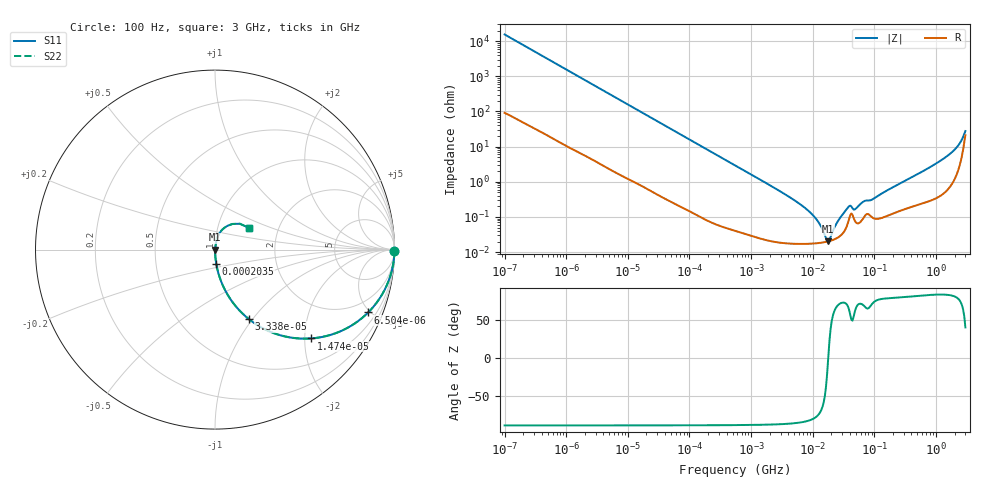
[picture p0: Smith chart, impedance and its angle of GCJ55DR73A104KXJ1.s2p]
!Murata Part Number: GCJ55DR73A104KXJ1
!These Parameters are Measured in Series Mode Connection
!Data Generated on Mar 13, 2026
!  o--ll--o
!Port1  Port2
!  o------o
!Operation Temp=25[degC], DC Bias Voltage=0[V]
!Freq. Start=100[Hz] Stop=3[GHz] 401[Steps]
# Hz S RI R 50
!Freq.(Hz) S11(Real) S11(Imag) S21(Real) S21(Imag) S12(Real) S12(Imag) S22(Real) S22(Imag)
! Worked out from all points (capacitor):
!   401 points, 100 Hz to 3 GHz, reference 50 ohm
!   read as one part in series: C = 103 nF near 109 Hz
!   lowest |Z| = 20.2 mohm at 17.89 MHz (marker M1)
!   series resonance near 17.83 MHz, so ESL is about 780 pH
!   S11 on the Smith chart (normalised r, x): 100 Hz: open; 6.504 kHz: 1.04, -4.86; 14.74 kHz: 1.02, -2.15; 33.38 kHz: 1.01, -0.95; 203.5 kHz: 1.00, -0.16; 3 GHz: 1.42, +0.36
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100  0.9999 -0.00645  7.96e-05 0.00645  7.96e-05 0.00645  0.9999 -0.00645
1788  0.9864 -0.1123  0.0136 0.1123  0.0136 0.1123  0.9864 -0.1123
6504  0.8532 -0.3503  0.1468 0.3503  0.1468 0.3503  0.8532 -0.3503
14736  0.5363 -0.4947  0.4637 0.4947  0.4637 0.4947  0.5363 -0.4947
31977  0.2006 -0.3964  0.7994 0.3964  0.7994 0.3964  0.2006 -0.3964
33383  0.1874 -0.3861  0.8126 0.3861  0.8126 0.3861  0.1874 -0.3861
69391  0.0521 -0.2179  0.9479 0.2179  0.9479 0.2179  0.0521 -0.2179
203529  0.00694 -0.0784  0.9931 0.0784  0.9931 0.0784  0.00694 -0.0784
547723  0.00127 -0.0294  0.9987 0.0294  0.9987 0.0294  0.00127 -0.0294
4323298  0.000187 -0.00355  0.9998 0.00355  0.9998 0.00355  0.000187 -0.00355
9794414  0.000176 -0.00117  0.9998 0.00117  0.9998 0.00117  0.000176 -0.00117
1.268047e7  0.000182 -0.000642  0.9998 0.000642  0.9998 0.000642  0.000182 -0.000642
1.789277e7  0.000202 6.4e-06  0.9998 -6.4e-06  0.9998 -6.4e-06  0.000202 6.4e-06
2.635803e7  0.000269 0.000778  0.9997 -0.000778  0.9997 -0.000778  0.000269 0.000778
3.71925e7  0.000674 0.00172  0.9993 -0.00172  0.9993 -0.00172  0.000674 0.00172
5.026954e7  0.000697 0.00159  0.9993 -0.00159  0.9993 -0.00159  0.000697 0.00159
6.794454e7  0.000996 0.00261  0.999 -0.00261  0.999 -0.00261  0.000996 0.00261
9.183415e7  0.000985 0.00296  0.999 -0.00296  0.999 -0.00296  0.000985 0.00296
1.751444e8  0.00117 0.00605  0.9988 -0.00605  0.9988 -0.00605  0.00117 0.00605
1.382454e9  0.00713 0.0471  0.9929 -0.0471  0.9929 -0.0471  0.00713 0.0471
2.126076e9  0.0224 0.0872  0.9776 -0.0872  0.9776 -0.0872  0.0224 0.0872
3e9  0.1918 0.12  0.8082 -0.12  0.8082 -0.12  0.1918 0.12
